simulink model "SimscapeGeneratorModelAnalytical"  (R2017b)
settings: Solver=VariableStepAuto  StartTime=0.0  StopTime=0.02  FixedStep=1e-5  RelTol=1e-3  AbsTol=1e-3  EnableMultiTasking=on
libraries: fl_lib x15, nesl_utility x12, pe_lib x2

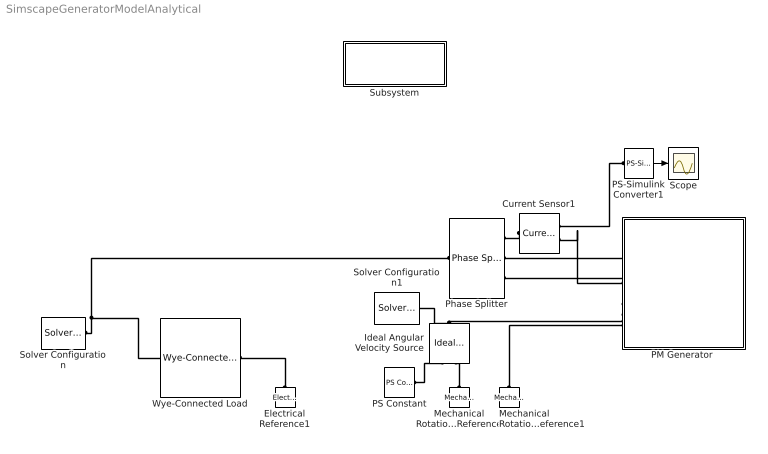
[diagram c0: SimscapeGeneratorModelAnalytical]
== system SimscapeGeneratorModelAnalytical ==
  Current Sensor1 : fl_lib/Electrical/Electrical Sensors/Current Sensor
  Electrical Reference1 : fl_lib/Electrical/Electrical Elements/Electrical Reference
  Ideal Angular Velocity Source : fl_lib/Mechanical/Mechanical Sources/Ideal Angular Velocity Source
  Mechanical Rotational Reference : fl_lib/Mechanical/Rotational Elements/Mechanical Rotational Reference
  Mechanical Rotational Reference1 : fl_lib/Mechanical/Rotational Elements/Mechanical Rotational Reference
  "PM Generator " : Subsystem
  PS Constant : fl_lib/Physical Signals/Sources/PS Constant  constant=2000*2*pi/60
  PS-Simulink Converter1 : nesl_utility/PS-Simulink Converter  PhysicalDomain=network_engine_domain  SubClassName=ps_output  LeftPortType=input  RightPortType=output  PseudoPeriodic=off  Frequencies=[]  Unit=1  AffineConversion=off
  Phase Splitter : pe_lib/Connections/Phase Splitter
  Scope : Scope
  Solver Configuration : nesl_utility/Solver Configuration  PhysicalDomain=network_engine_domain  SubClassName=solver  LeftPortType=input  RightPortType=generic  Accelerate=off  Tones=[]  Harmonics=[]  SimulateNoise=off  Profile=off  UseLocalSampling=off  EnableSwitchedLinearOptims=on  FrequencyDomain=off  UseCCode=off  RelTol=0.001  AbsTol=1e-06  MinStep=1e-09  ToWorkspace=off  RevertToSquareIcSolve=off  NumHomotopyIterations=100  PhasorMode=off  PhasorModeNumHarmonics=1  DoDC=off  ResidualTolerance=1e-09  UseLocalSolver=off  LocalSolverChoice=NE_BACKWARD_EULER_ADVANCER  LocalSolverSampleTime=0.001  DoFixedCost=off  MaxNonlinIter=3  MaxModeIter=2  LinearAlgebra=Sparse  DelaysMemoryBudget=1024  AutomaticFiltering=on  FilteringTimeConstant=0.001
  Solver Configuration1 : nesl_utility/Solver Configuration  PhysicalDomain=network_engine_domain  SubClassName=solver  LeftPortType=input  RightPortType=generic  Accelerate=off  Tones=[]  Harmonics=[]  SimulateNoise=off  Profile=off  UseLocalSampling=off  EnableSwitchedLinearOptims=on  FrequencyDomain=off  UseCCode=off  RelTol=0.001  AbsTol=1e-06  MinStep=1e-09  ToWorkspace=off  RevertToSquareIcSolve=off  NumHomotopyIterations=100  PhasorMode=off  PhasorModeNumHarmonics=1  DoDC=off  ResidualTolerance=1e-09  UseLocalSolver=off  LocalSolverChoice=NE_BACKWARD_EULER_ADVANCER  LocalSolverSampleTime=0.001  DoFixedCost=off  MaxNonlinIter=3  MaxModeIter=2  LinearAlgebra=Sparse  DelaysMemoryBudget=1024  AutomaticFiltering=on  FilteringTimeConstant=0.001
  Subsystem : Subsystem
  Wye-Connected Load : pe_lib/Passive Devices/Wye-Connected Load  parameterization=1  component_structure=1  component_structure_PQ=1  R=6.6 Ohm  L=0.001 H  C=1e-6 F  IL0=[ 0 0 0 ] A  VC0=[ 0 0 0 ] V  R_parasitic=1e-6 Ohm  G_parasitic=1e-6 1/Ohm  VRated=2.4e+4 V  FRated=60 Hz  P=1000 W  Qpos=100 V*A  Qneg=-100 V*A  Vmag0=2.4e+4 V  Vang0=0 deg  Freq0=60 Hz  R_parasitic_PQ=1e-6 Ohm  G_parasitic_PQ=1e-6 1/Ohm
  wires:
  PS-Simulink Converter1/1 -> Scope/1
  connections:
  "PM Generator "/LConn2 -- Phase Splitter/RConn2
  "PM Generator "/LConn3 -- Phase Splitter/RConn3
  Solver Configuration/RConn1 -- Wye-Connected Load/LConn1 -- Phase Splitter/LConn1
  PS-Simulink Converter1/LConn1 -- Current Sensor1/RConn1
  Mechanical Rotational Reference/LConn1 -- Ideal Angular Velocity Source/RConn2
  Ideal Angular Velocity Source/LConn1 -- "PM Generator "/LConn4 -- Solver Configuration1/RConn1
  Mechanical Rotational Reference1/LConn1 -- "PM Generator "/LConn5
  PS Constant/RConn1 -- Ideal Angular Velocity Source/RConn1
  Current Sensor1/RConn2 -- "PM Generator "/LConn1
  Electrical Reference1/LConn1 -- Wye-Connected Load/RConn1
  Current Sensor1/LConn1 -- Phase Splitter/RConn1

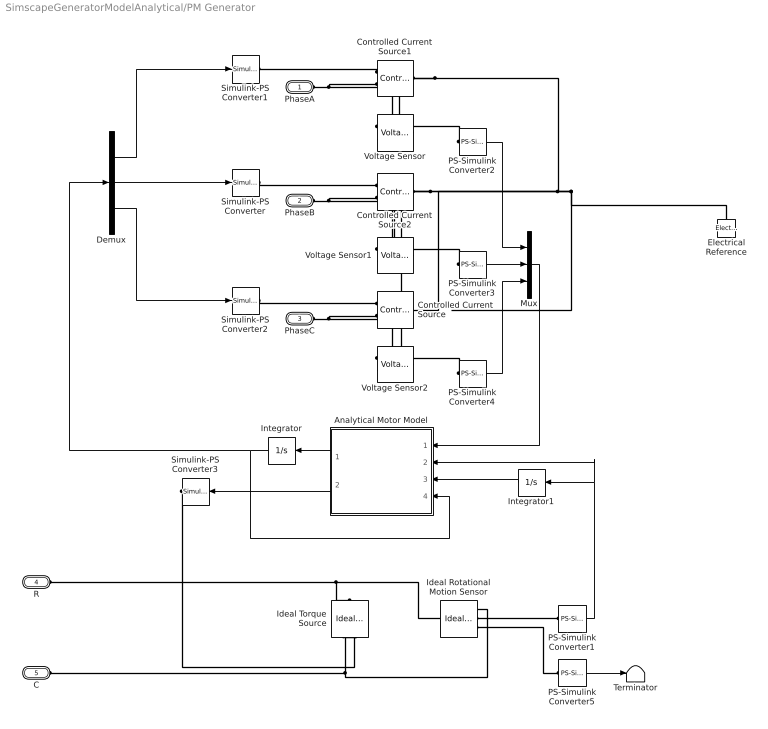
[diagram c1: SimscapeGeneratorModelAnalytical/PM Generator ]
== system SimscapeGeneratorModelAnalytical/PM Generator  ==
  Analytical Motor Model : Subsystem
  Controlled Current Source : fl_lib/Electrical/Electrical Sources/Controlled Current Source
  Controlled Current Source1 : fl_lib/Electrical/Electrical Sources/Controlled Current Source
  Controlled Current Source2 : fl_lib/Electrical/Electrical Sources/Controlled Current Source
  Demux : Demux  Outputs=3
  Electrical Reference : fl_lib/Electrical/Electrical Elements/Electrical Reference
  Ideal Rotational Motion Sensor : fl_lib/Mechanical/Mechanical Sensors/Ideal Rotational Motion Sensor  offset=0 rad
  Ideal Torque Source : fl_lib/Mechanical/Mechanical Sources/Ideal Torque Source
  Integrator : Integrator
  Integrator1 : Integrator
  Mux : Mux  Inputs=3
  PS-Simulink Converter{1..5} (5 alike) : nesl_utility/PS-Simulink Converter  PhysicalDomain=network_engine_domain  SubClassName=ps_output  LeftPortType=input  RightPortType=output  PseudoPeriodic=off  Frequencies=[]  Unit=1  AffineConversion=off
  Simulink-PS Converter{,1..3} (4 alike) : nesl_utility/Simulink-PS Converter  PhysicalDomain=network_engine_domain  SubClassName=ps_input  LeftPortType=input  RightPortType=output  PseudoPeriodic=off  Frequencies=[]  NoiseDistribution=none  NoiseParameters=[]  Unit=1  AffineConversion=off  FilteringAndDerivatives=zero  SimscapeFilterOrder=1  InputFilterTimeConstant=0.001  UdotUserProvided=1
  Terminator : Terminator
  Voltage Sensor : fl_lib/Electrical/Electrical Sensors/Voltage Sensor
  Voltage Sensor1 : fl_lib/Electrical/Electrical Sensors/Voltage Sensor
  Voltage Sensor2 : fl_lib/Electrical/Electrical Sensors/Voltage Sensor
  PhaseA : PMIOPort  Port=1  Side=Left
  PhaseB : PMIOPort  Port=2  Side=Left
  PhaseC : PMIOPort  Port=3  Side=Left
  R : PMIOPort  Port=4  Side=Left
  C : PMIOPort  Port=5  Side=Left
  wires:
  Analytical Motor Model/1(dxdt) -> Integrator/1
  Mux/1 -> Analytical Motor Model/1(u)
  Integrator/1 -> Analytical Motor Model/4(x), Demux/1
  PS-Simulink Converter3/1 -> Mux/2
  PS-Simulink Converter4/1 -> Mux/3
  PS-Simulink Converter2/1 -> Mux/1
  Demux/2 -> Simulink-PS Converter/1
  Demux/1 -> Simulink-PS Converter1/1
  Demux/3 -> Simulink-PS Converter2/1
  PS-Simulink Converter1/1 -> Analytical Motor Model/2(omega), Integrator1/1
  PS-Simulink Converter5/1 -> Terminator/1
  Integrator1/1 -> Analytical Motor Model/3(tta)
  Analytical Motor Model/2(tq) -> Simulink-PS Converter3/1
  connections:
  PhaseA/RConn1 -- Voltage Sensor/LConn1 -- Controlled Current Source1/RConn2
  PhaseB/RConn1 -- Voltage Sensor1/LConn1 -- Controlled Current Source2/RConn2
  PhaseC/RConn1 -- Voltage Sensor2/LConn1 -- Controlled Current Source/RConn2
  PS-Simulink Converter2/LConn1 -- Voltage Sensor/RConn1
  PS-Simulink Converter3/LConn1 -- Voltage Sensor1/RConn1
  PS-Simulink Converter4/LConn1 -- Voltage Sensor2/RConn1
  Simulink-PS Converter/RConn1 -- Controlled Current Source2/RConn1
  Simulink-PS Converter2/RConn1 -- Controlled Current Source/RConn1
  Controlled Current Source1/RConn1 -- Simulink-PS Converter1/RConn1
  C/RConn1 -- Ideal Rotational Motion Sensor/RConn1 -- Ideal Torque Source/RConn2
  R/RConn1 -- Ideal Torque Source/LConn1 -- Ideal Rotational Motion Sensor/LConn1
  Simulink-PS Converter3/RConn1 -- Ideal Torque Source/RConn1
  PS-Simulink Converter1/LConn1 -- Ideal Rotational Motion Sensor/RConn2
  PS-Simulink Converter5/LConn1 -- Ideal Rotational Motion Sensor/RConn3
  Controlled Current Source1/LConn1 -- Voltage Sensor/RConn2 -- Electrical Reference/LConn1 -- Voltage Sensor2/RConn2 -- Controlled Current Source/LConn1 -- Voltage Sensor1/RConn2 -- Controlled Current Source2/LConn1

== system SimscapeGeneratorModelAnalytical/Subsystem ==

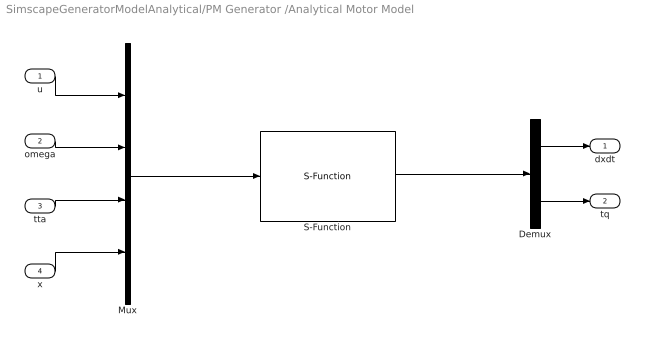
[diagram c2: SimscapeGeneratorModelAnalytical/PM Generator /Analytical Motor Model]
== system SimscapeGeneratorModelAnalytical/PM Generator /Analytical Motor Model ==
  u : Inport
  omega : Inport  Port=2
  tta : Inport  Port=3
  x : Inport  Port=4
  Demux : Demux  Outputs=[3 1]
  Mux : Mux  Inputs=[3 1 1 3]
  S-Function : S-Function  FunctionName=MotorModelAnalytical  SFunctionDeploymentMode=off  EnableBusSupport=off
  dxdt : Outport
  tq : Outport  Port=2
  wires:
  u/1 -> Mux/1
  omega/1 -> Mux/2
  tta/1 -> Mux/3
  x/1 -> Mux/4
  Demux/1 -> dxdt/1
  Demux/2 -> tq/1
  S-Function/1 -> Demux/1
  Mux/1 -> S-Function/1
